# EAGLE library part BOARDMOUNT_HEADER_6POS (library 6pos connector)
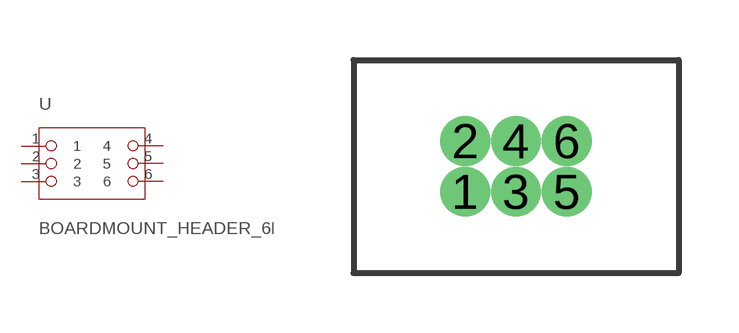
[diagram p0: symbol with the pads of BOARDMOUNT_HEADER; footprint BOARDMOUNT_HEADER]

Designator prefix -

## BOARDMOUNT_HEADER_6POS  [BOARDMOUNT_HEADER]
1  1
2  2
3  3
4  4
5  5
6  6

## Footprint BOARDMOUNT_HEADER (pad centres in mm)
drill 0.737: 1 -1.27,-1.27; 2 -1.27,0; 3 0,-1.27; 4 0,0; 5 1.27,-1.27; 6 1.27,0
